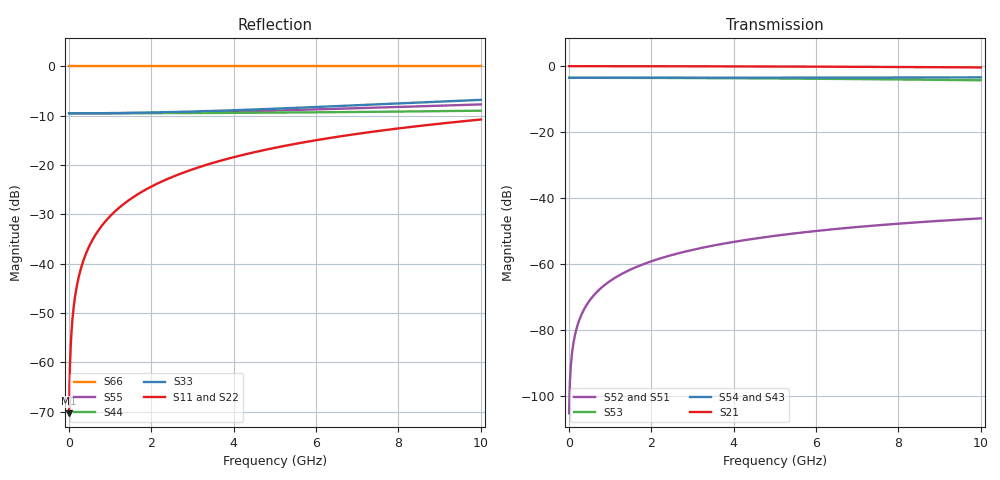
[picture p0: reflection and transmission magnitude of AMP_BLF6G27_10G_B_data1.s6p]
! Created Fri Aug 20 16:12:58 2010
# ghz S ma R 50
! 6 Port Network Data from SP1.SP block
! freq  magS11  angS11  magS12  angS12  magS13  angS13  magS14  angS14
!  magS15  angS15  magS16  angS16
!  magS21  angS21  magS22  angS22
!  magS23  angS23  magS24  angS24  magS25  angS25  magS26  angS26
!  magS31  angS31  magS32  angS32  magS33  angS33  magS34  angS34
!  magS35  angS35  magS36  angS36
!  magS41  angS41  magS42  angS42
!  magS43  angS43  magS44  angS44  magS45  angS45  magS46  angS46
!  magS51  angS51  magS52  angS52  magS53  angS53  magS54  angS54
!  magS55  angS55  magS56  angS56
!  magS61  angS61  magS62  angS62
!  magS63  angS63  magS64  angS64  magS65  angS65  magS66  angS66
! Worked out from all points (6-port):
!   1000 points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, 10 MHz to 10 GHz, reference 50 ohm
!   strongest paths, dB at 10 MHz, 2.51 GHz, 5.01 GHz, 7.51 GHz, 10 GHz:
!     S21: 0.0, 0.0, -0.1, -0.2, -0.4
!     S54: -3.5, -3.5, -3.5, -3.4, -3.4
!     S43: -3.5, -3.5, -3.6, -3.7, -3.8
!     S53: -3.5, -3.6, -3.7, -4.0, -4.3
!     S52: -105.3, -57.3, -51.4, -48.2, -46.2
!     S51: -105.3, -57.3, -51.4, -48.2, -46.2
!   lowest |S11| = -70.3 dB at 10 MHz (marker M1), VSWR 1.00, Z = 50 + j0.0301 ohm
!   |S11| at or under -10 dB: start of sweep to end of sweep
